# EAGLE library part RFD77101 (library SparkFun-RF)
Simblee  BLE Module RFD77101 © 2015 RF Digital Corporation Datasheet PATENTS PENDING 04.01.2015 Bluetooth Smart radio transceiver, ARM Cortex M0 microcontroller. 128kB Flash, 24kB RAM, no EEPROM Arduino-compatible. SparkFun Products: Simblee BLE Module - RFD77101 SparkFun Simblee BLE Breakout - RFD77101
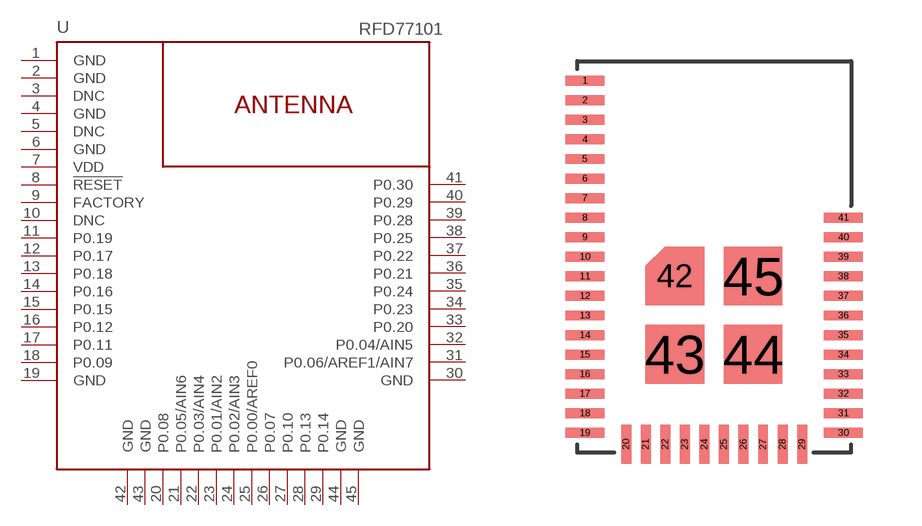
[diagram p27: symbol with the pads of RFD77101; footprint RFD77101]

Designator prefix U

## RFD77101 (PROD_ID: COMP-13237; SF_ID: WRL-13808)  [RFD77101]
1  GND  pwr
2  GND  pwr
3  DNC  nc
4  GND  pwr
5  DNC  nc
6  GND  pwr
7  VDD  pwr
8  !RESET!  in
9  FACTORY  nc
10  DNC  nc
11  P0.19
12  P0.17
13  P0.18
14  P0.16
15  P0.15
16  P0.12
17  P0.11
18  P0.09
19  GND  pwr
20  P0.08
21  P0.05/AIN6
22  P0.03/AIN4
23  P0.01/AIN2
24  P0.02/AIN3
25  P0.00/AREF0
26  P0.07
27  P0.10
28  P0.13
29  P0.14
30  GND  pwr
31  P0.06/AREF1/AIN7
32  P0.04/AIN5
33  P0.20
34  P0.23
35  P0.24
36  P0.21
37  P0.22
38  P0.25
39  P0.28
40  P0.29
41  P0.30
42  GND  pwr
43  GND  pwr
44  GND  pwr
45  GND  pwr

## Footprint RFD77101 (pad centres in mm)
Simblee  BLE Module RFD77101 © 2015 RF Digital Corporation www.RFDigital.com www.Simblee.com PATENTS PENDING 04.01.2015 Specifications: Pin count: 45 Pin pitch:0.5mm Area:7mmx10mm Datasheet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
smd 1 x 0.254: 1 0,0; 2 0,-0.5; 3 0,-1; 4 0,-1.5; 5 0,-2; 6 0,-2.5; 7 0,-3; 8 0,-3.5; 9 0,-4; 10 0,-4.5; 11 0,-5; 12 0,-5.5; 13 0,-6; 14 0,-6.5; 15 0,-7; 16 0,-7.5; 17 0,-8; 18 0,-8.5; 19 0,-9; 30 6.61,-9; 31 6.61,-8.5; 32 6.61,-8; 33 6.61,-7.5; 34 6.61,-7; 35 6.61,-6.5; 36 6.61,-6; 37 6.61,-5.5; 38 6.61,-5; 39 6.61,-4.5; 40 6.61,-4; 41 6.61,-3.5
smd 0.254 x 1: 20 1.055,-9.29; 21 1.555,-9.29; 22 2.055,-9.29; 23 2.555,-9.29; 24 3.055,-9.29; 25 3.555,-9.29; 26 4.055,-9.29; 27 4.555,-9.29; 28 5.055,-9.29; 29 5.555,-9.29
smd 0.9 x 0.9: 42 2.3,-4.99
smd 1.5 x 1.5: 43 2.3,-6.99; 44 4.3,-6.99; 45 4.3,-4.99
